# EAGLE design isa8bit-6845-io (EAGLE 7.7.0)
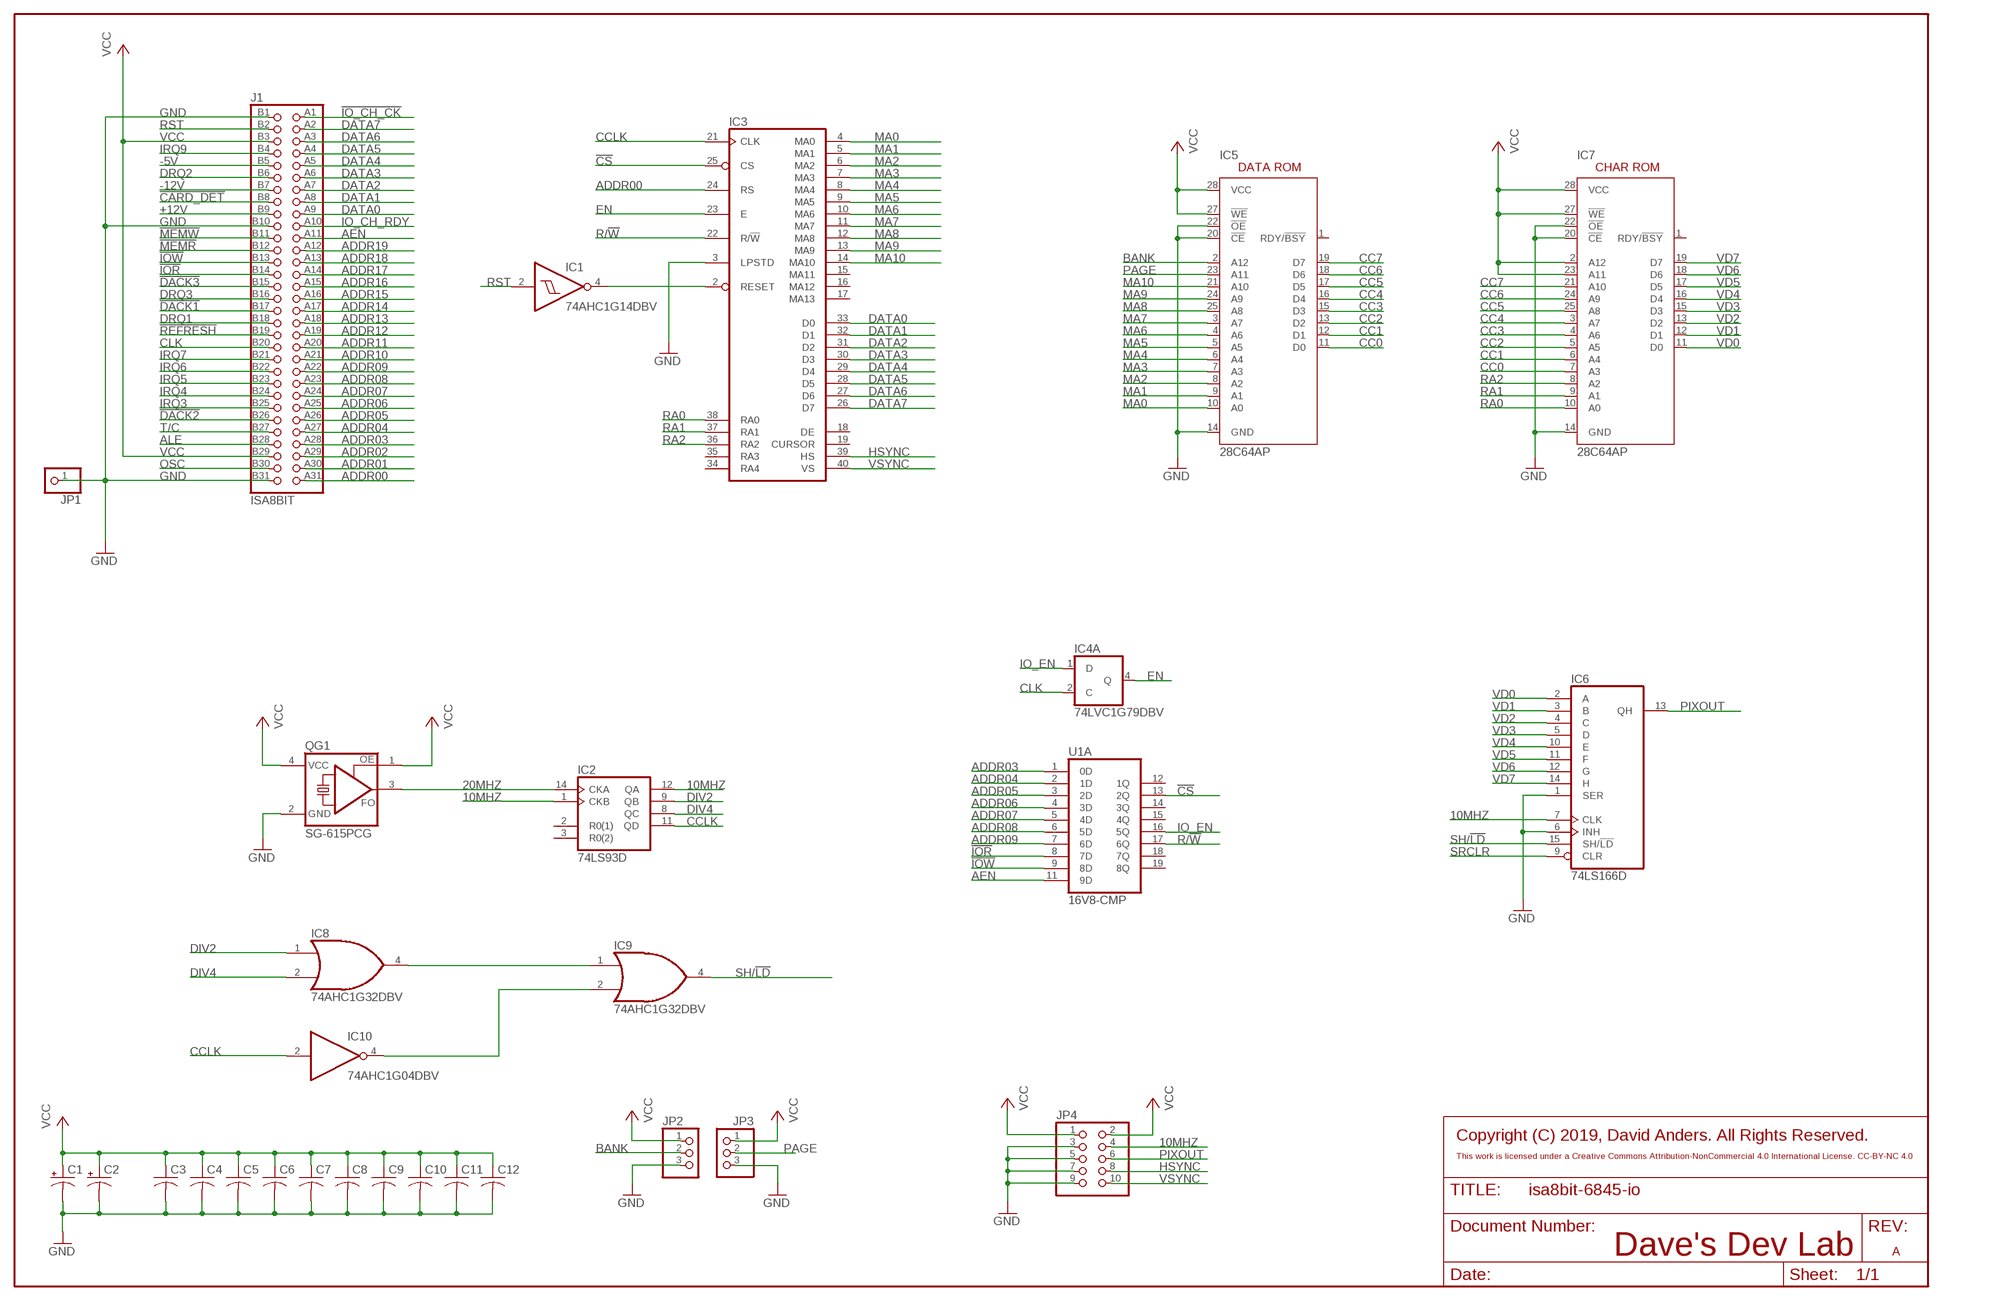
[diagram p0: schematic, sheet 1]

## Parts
C1  CPOL-USTT2D5  [TT2D5]
C2  CPOL-USTT2D5  [TT2D5]
C3  C-USC0603  [C0603]
C4  C-USC0603  [C0603]
C5  C-USC0603  [C0603]
C6  C-USC0603  [C0603]
C7  C-USC0603  [C0603]
C8  C-USC0603  [C0603]
C9  C-USC0603  [C0603]
C10  C-USC0603  [C0603]
C11  C-USC0603  [C0603]
C12  C-USC0603  [C0603]
IC1  74AHC1G14DBV  [SOT23-5]
IC2  74LS93D  [SO14]
IC3  6845  [DIL40]
IC4  74LVC1G79DBV  [SOT23-5]
IC5  28C64AP  [DIL28-6]
IC6  74LS166D  [SO16]
IC7  28C64AP  [DIL28-6]
IC8  74AHC1G32DBV  [SOT23-5]
IC9  74AHC1G32DBV  [SOT23-5]
IC10  74AHC1G04DBV  [SOT23-5]
J1  ISA8BIT  [ISA8BIT-LARGE]
JP1  PINHD-1X1  [1X01]
JP2  PINHD-1X3  [1X03]
JP3  PINHD-1X3  [1X03]
JP4  PINHD-2X5  [2X05]
QG1  SG-615PCG  [SG-615]
U1  16V8-CMP  [DIL20]

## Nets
10MHZ: IC2.1(CKB) IC2.12(QA) IC6.7(CLK) JP4.4
20MHZ: IC2.14(CKA) QG1.3(FO)
!CARD_DET: J1.B8
!CS: IC3.25(CS) U1.13(A:2Q)
!DACK1: J1.B17
!DACK2: J1.B26
!DACK3: J1.B15
!IO_CH_CK: J1.A1
!IOR: J1.B14 U1.8(A:7D)
!IOW: J1.B13 U1.9(A:8D)
!MEMR: J1.B12
!MEMW: J1.B11
!REFRESH: J1.B19
+12V: J1.B9
-5V: J1.B5
-12V: J1.B7
ADDR00: IC3.24(RS) J1.A31
ADDR01: J1.A30
ADDR02: J1.A29
ADDR03: J1.A28 U1.1(A:0D)
ADDR04: J1.A27 U1.2(A:1D)
ADDR05: J1.A26 U1.3(A:2D)
ADDR06: J1.A25 U1.4(A:3D)
ADDR07: J1.A24 U1.5(A:4D)
ADDR08: J1.A23 U1.6(A:5D)
ADDR09: J1.A22 U1.7(A:6D)
ADDR10: J1.A21
ADDR11: J1.A20
ADDR12: J1.A19
ADDR13: J1.A18
ADDR14: J1.A17
ADDR15: J1.A16
ADDR16: J1.A15
ADDR17: J1.A14
ADDR18: J1.A13
ADDR19: J1.A12
AEN: J1.A11 U1.11(A:9D)
ALE: J1.B28
BANK: IC5.2(A12) JP2.2
CC0: IC5.11(D0) IC7.7(A3)
CC1: IC5.12(D1) IC7.6(A4)
CC2: IC5.13(D2) IC7.5(A5)
CC3: IC5.15(D3) IC7.4(A6)
CC4: IC5.16(D4) IC7.3(A7)
CC5: IC5.17(D5) IC7.25(A8)
CC6: IC5.18(D6) IC7.24(A9)
CC7: IC5.19(D7) IC7.21(A10)
CCLK: IC2.11(QD) IC3.21(CLK) IC10.2(I)
CLK: IC4.2(C) J1.B20
DATA0: IC3.33(D0) J1.A9
DATA1: IC3.32(D1) J1.A8
DATA2: IC3.31(D2) J1.A7
DATA3: IC3.30(D3) J1.A6
DATA4: IC3.29(D4) J1.A5
DATA5: IC3.28(D5) J1.A4
DATA6: IC3.27(D6) J1.A3
DATA7: IC3.26(D7) J1.A2
DIV2: IC2.9(QB) IC8.1(I0)
DIV4: IC2.8(QC) IC8.2(I1)
DRQ1: J1.B18
DRQ2: J1.B6
DRQ3: J1.B16
EN: IC3.23(E) IC4.4(Q)
GND: C1.- C2.- C3.2 C4.2 C5.2 C6.2 C7.2 C8.2 C9.2 C10.2 C11.2 C12.2 IC3.3(LPSTD) IC5.14(GND) IC5.20(!CE) IC5.22(!OE) IC6.1(SER) IC6.6(INH) IC7.14(GND) IC7.20(!CE) IC7.22(!OE) J1.B1 J1.B10 J1.B31 JP1.1 JP2.3 JP3.3 JP4.3 JP4.5 JP4.7 JP4.9 QG1.2(GND)
HSYNC: IC3.39(HS) JP4.8
IO_CH_RDY: J1.A10
IO_EN: IC4.1(D) U1.16(A:5Q)
IRQ3: J1.B25
IRQ4: J1.B24
IRQ5: J1.B23
IRQ6: J1.B22
IRQ7: J1.B21
IRQ9: J1.B4
MA0: IC3.4(MA0) IC5.10(A0)
MA1: IC3.5(MA1) IC5.9(A1)
MA2: IC3.6(MA2) IC5.8(A2)
MA3: IC3.7(MA3) IC5.7(A3)
MA4: IC3.8(MA4) IC5.6(A4)
MA5: IC3.9(MA5) IC5.5(A5)
MA6: IC3.10(MA6) IC5.4(A6)
MA7: IC3.11(MA7) IC5.3(A7)
MA8: IC3.12(MA8) IC5.25(A8)
MA9: IC3.13(MA9) IC5.24(A9)
MA10: IC3.14(MA10) IC5.21(A10)
N$1: IC8.4(O) IC9.1(I0)
N$2: IC1.4(O) IC3.2(RESET)
N$4: IC9.2(I1) IC10.4(O)
OSC: J1.B30
PAGE: IC5.23(A11) JP3.2
PIXOUT: IC6.13(QH) JP4.6
R/!W: IC3.22(R/!W) U1.17(A:6Q)
RA0: IC3.38(RA0) IC7.10(A0)
RA1: IC3.37(RA1) IC7.9(A1)
RA2: IC3.36(RA2) IC7.8(A2)
RST: IC1.2(I) J1.B2
SH/!LD: IC6.15(SH/!LD) IC9.4(O)
SRCLR: IC6.9(CLR)
T/C: J1.B27
VCC: C1.+ C2.+ C3.1 C4.1 C5.1 C6.1 C7.1 C8.1 C9.1 C10.1 C11.1 C12.1 IC5.27(!WE) IC5.28(VCC) IC7.2(A12) IC7.23(A11) IC7.27(!WE) IC7.28(VCC) J1.B3 J1.B29 JP2.1 JP3.1 JP4.1 JP4.2 QG1.1(OE) QG1.4(VCC)
VD0: IC6.2(A) IC7.11(D0)
VD1: IC6.3(B) IC7.12(D1)
VD2: IC6.4(C) IC7.13(D2)
VD3: IC6.5(D) IC7.15(D3)
VD4: IC6.10(E) IC7.16(D4)
VD5: IC6.11(F) IC7.17(D5)
VD6: IC6.12(G) IC7.18(D6)
VD7: IC6.14(H) IC7.19(D7)
VSYNC: IC3.40(VS) JP4.10
Unconnected: IC2.2(R0(1)) IC2.3(R0(2)) IC3.15(MA11) IC3.16(MA12) IC3.17(MA13) IC3.18(DE) IC3.19(CURSOR) IC3.34(RA4) IC3.35(RA3) IC5.1(RDY/!BSY) IC7.1(RDY/!BSY) U1.12(A:1Q) U1.14(A:3Q) U1.15(A:4Q) U1.18(A:7Q) U1.19(A:8Q)

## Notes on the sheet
- DATA ROM | CHAR ROM
- Copyright (C) 2019, David Anders. All Rights Reserved.
- This work is licensed under a Creative Commons Attribution-NonCommercial 4.0 International License. CC-BY-NC 4.0
- Dave's Dev Lab | A

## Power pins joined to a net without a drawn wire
GND: IC1.3(GND) IC2.10(GND) IC3.1(GND) IC4.3(GND) IC6.8(GND) IC8.3(GND) IC9.3(GND) IC10.3(GND) U1.10(B:GND)
VCC: IC1.5(VCC) IC2.5(VCC) IC3.20(VCC) IC4.5(VCC) IC6.16(VCC) IC8.5(VCC) IC9.5(VCC) IC10.5(VCC) U1.20(B:VCC)

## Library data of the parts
C1 C2 = resistor:CPOL-US: POLARIZED CAPACITOR, American symbol
C3-C12 = resistor:C-US: CAPACITOR, American symbol
IC1 = 74xx-little-us:74*1G14: Single Schmitt-Trigger Inverter Gate
IC2 = 74xx-us:74*93: Decade, divide by twelve and binary COUNTER
IC3 = micro-motorola:6845: MICROCONTROLLER/MEMORY DEVICE; OC_FARNELL: unknown; OC_NEWARK: unknown
IC4 = 74xx-little-us:74*1G79: Single Positive-Edge-Triggered D-Type Flip-Flop Source: Data sheet
IC5 IC7 = microchip:28*64A: CMOS EEPROM 64 K (8 K x 8), low voltage; MPN: AT28C64B-15PU; OC_FARNELL: 1631144; OC_NEWARK: 96K6557
IC6 = 74xx-us:74*166: 8-bit parallel load SHIFT REGISTER
IC8 IC9 = 74xx-little-us:74*1G32: 2-input OR gate
IC10 = 74xx-little-us:74*1G04: INVERTER Gate
J1 = custom-misc:ISA8BIT
JP1 = custom-pinhead:PINHD-1X1: PIN HEADER
JP2 JP3 = custom-pinhead:PINHD-1X3: PIN HEADER
JP4 = custom-pinhead:PINHD-2X5: PIN HEADER
QG1 = crystal:SG-615: SOJ HIGH-FREQUENCY CRYSTAL OSCILLATOR Source: Crystal Oscillator SG-615%20Series.pdf; MPN: SG615P-50MHZ 50PPM; OC_FARNELL: 1216207; OC_NEWARK: 01M8855
U1 = custom-misc:16V8-CMP

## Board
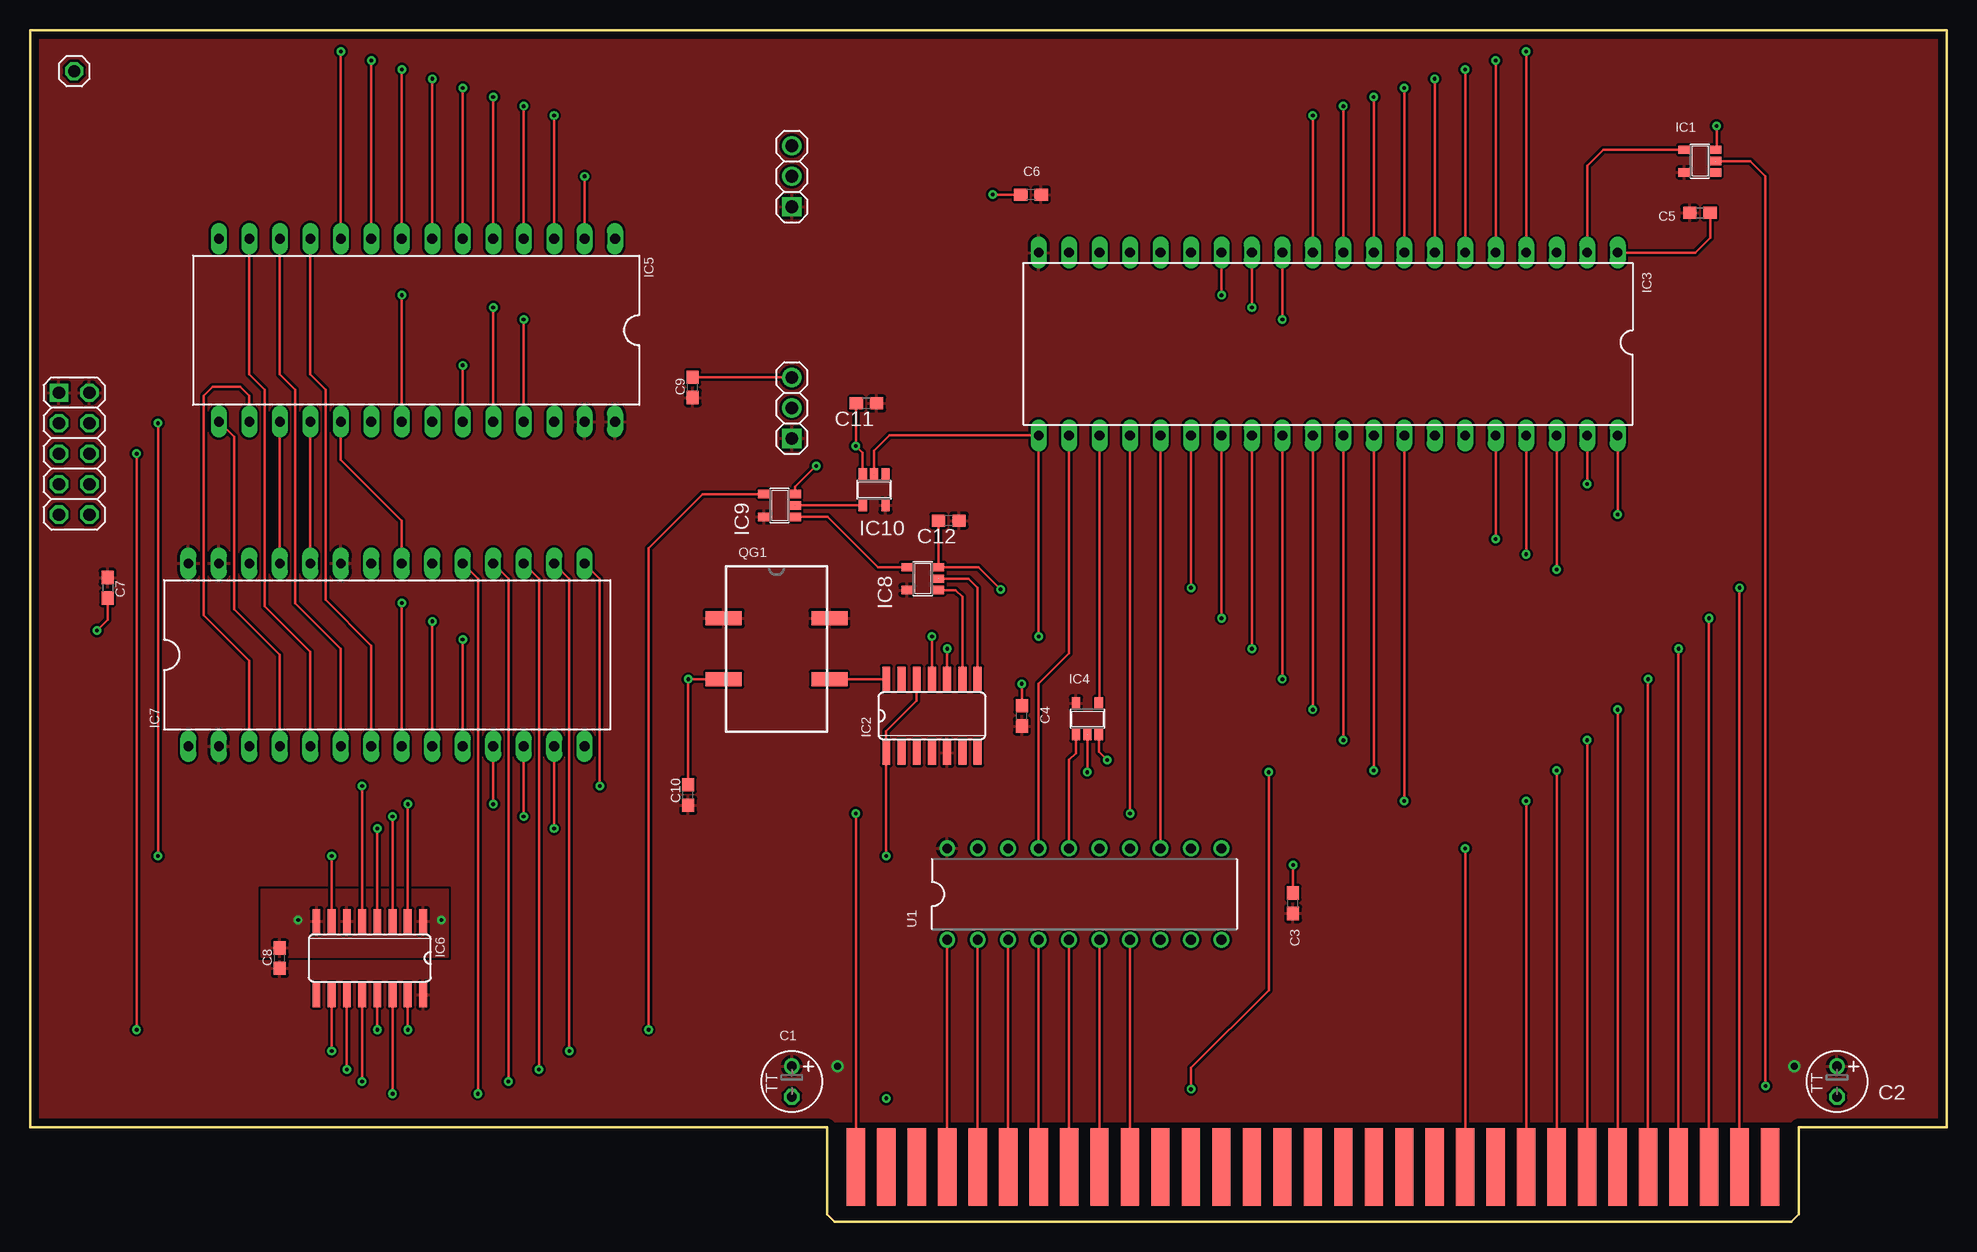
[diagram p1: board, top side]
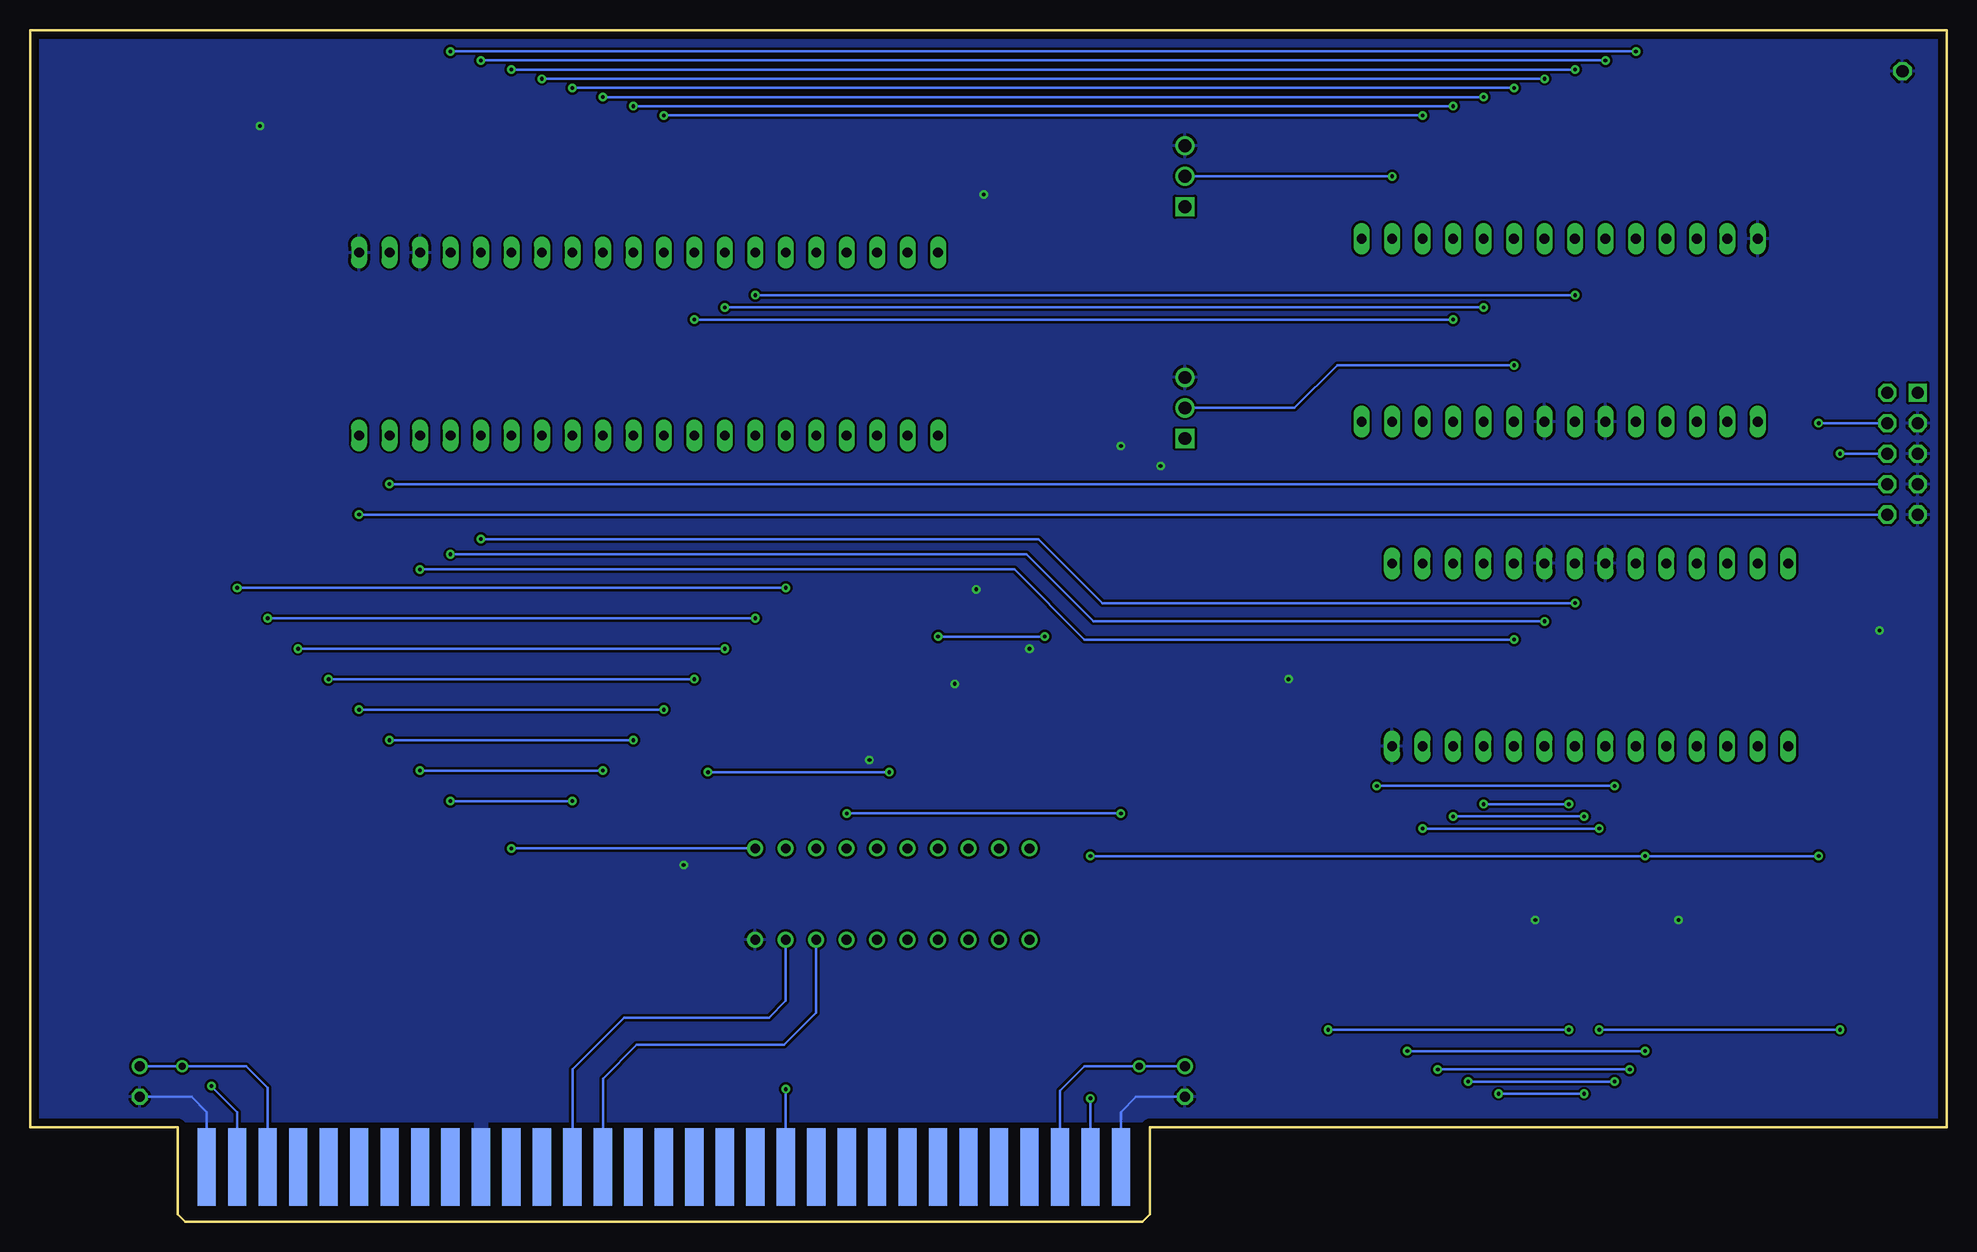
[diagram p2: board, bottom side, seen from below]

Size 159.77 x 99.31 mm. Coordinates in mm from the lower left corner, seen from the top.
Copper layers (1*16): Top 0.035mm / dielectric 1.5mm / Bottom 0.035mm
Design rules "default *": minimum track width 8mil, minimum drill 12mil, track to track 8mil, track to pad 8mil, pad to pad 8mil, via to via 8mil, smd to smd 8mil, copper to edge 25mil, drill to drill 8mil, minimum pad ring 10mil, minimum via ring 8mil, stop-mask expansion 4mil, vias tented up to drill 0mil, thermal gap 10mil

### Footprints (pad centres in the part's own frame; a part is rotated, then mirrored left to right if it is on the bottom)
TT2D5 = drill 0.813: + -1.27,0 | drill 0.813 octagon: - 1.27,0
C0603 = smd 1.1 x 1: 1 -0.85,0; 2 0.85,0
SOT23-5 = smd 0.69 x 0.99: 1 -0.95,-1.29; 2 0,-1.29; 3 0.95,-1.29; 4 0.95,1.3; 5 -0.95,1.3
SO14 = smd 0.66 x 2.032: 1 -3.81,-3.073; 2 -2.54,-3.073; 3 -1.27,-3.073; 4 0,-3.073; 5 1.27,-3.073; 6 2.54,-3.073; 7 3.81,-3.073; 8 3.81,3.073; 9 2.54,3.073; 10 1.27,3.073; 11 0,3.073; 12 -1.27,3.073; 13 -2.54,3.073; 14 -3.81,3.073
DIL40 = drill 0.813 long: 1 -24.13,-7.62; 2 -21.59,-7.62; 3 -19.05,-7.62; 4 -16.51,-7.62; 5 -13.97,-7.62; 6 -11.43,-7.62; 7 -8.89,-7.62; 8 -6.35,-7.62; 9 -3.81,-7.62; 10 -1.27,-7.62; 11 1.27,-7.62; 12 3.81,-7.62; 13 6.35,-7.62; 14 8.89,-7.62; 15 11.43,-7.62; 16 13.97,-7.62; 17 16.51,-7.62; 18 19.05,-7.62; 19 21.59,-7.62; 20 24.13,-7.62; 21 24.13,7.62; 22 21.59,7.62; 23 19.05,7.62; 24 16.51,7.62; 25 13.97,7.62; 26 11.43,7.62; 27 8.89,7.62; 28 6.35,7.62; 29 3.81,7.62; 30 1.27,7.62; 31 -1.27,7.62; 32 -3.81,7.62; 33 -6.35,7.62; 34 -8.89,7.62; 35 -11.43,7.62; 36 -13.97,7.62; 37 -16.51,7.62; 38 -19.05,7.62; 39 -21.59,7.62; 40 -24.13,7.62
DIL28-6 = drill 0.813 long: 1 -16.51,-7.62; 2 -13.97,-7.62; 3 -11.43,-7.62; 4 -8.89,-7.62; 5 -6.35,-7.62; 6 -3.81,-7.62; 7 -1.27,-7.62; 8 1.27,-7.62; 9 3.81,-7.62; 10 6.35,-7.62; 11 8.89,-7.62; 12 11.43,-7.62; 13 13.97,-7.62; 14 16.51,-7.62; 15 16.51,7.62; 16 13.97,7.62; 17 11.43,7.62; 18 8.89,7.62; 19 6.35,7.62; 20 3.81,7.62; 21 1.27,7.62; 22 -1.27,7.62; 23 -3.81,7.62; 24 -6.35,7.62; 25 -8.89,7.62; 26 -11.43,7.62; 27 -13.97,7.62; 28 -16.51,7.62
SO16 = smd 0.66 x 2.032: 1 -4.445,-3.073; 2 -3.175,-3.073; 3 -1.905,-3.073; 4 -0.635,-3.073; 5 0.635,-3.073; 6 1.905,-3.073; 7 3.175,-3.073; 8 4.445,-3.073; 9 4.445,3.073; 10 3.175,3.073; 11 1.905,3.073; 12 0.635,3.073; 13 -0.635,3.073; 14 -1.905,3.073; 15 -3.175,3.073; 16 -4.445,3.073
ISA8BIT-LARGE = smd 1.524 x 6.477: A1 145.034,5.08; A2 142.494,5.08; A3 139.954,5.08; A4 137.414,5.08; A5 134.874,5.08; A6 132.334,5.08; A7 129.794,5.08; A8 127.254,5.08; A9 124.714,5.08; A10 122.174,5.08; A11 119.634,5.08; A12 117.094,5.08; A13 114.554,5.08; A14 112.014,5.08; A15 109.474,5.08; A16 106.934,5.08; A17 104.394,5.08; A18 101.854,5.08; A19 99.314,5.08; A20 96.774,5.08; A21 94.234,5.08; A22 91.694,5.08; A23 89.154,5.08; A24 86.614,5.08; A25 84.074,5.08; A26 81.534,5.08; A27 78.994,5.08; A28 76.454,5.08; A29 73.914,5.08; A30 71.374,5.08; A31 68.834,5.08 | smd 1.524 x 6.477 bottom: B1 145.034,5.08; B2 142.494,5.08; B3 139.954,5.08; B4 137.414,5.08; B5 134.874,5.08; B6 132.334,5.08; B7 129.794,5.08; B8 127.254,5.08; B9 124.714,5.08; B10 122.174,5.08; B11 119.634,5.08; B12 117.094,5.08; B13 114.554,5.08; B14 112.014,5.08; B15 109.474,5.08; B16 106.934,5.08; B17 104.394,5.08; B18 101.854,5.08; B19 99.314,5.08; B20 96.774,5.08; B21 94.234,5.08; B22 91.694,5.08; B23 89.154,5.08; B24 86.614,5.08; B25 84.074,5.08; B26 81.534,5.08; B27 78.994,5.08; B28 76.454,5.08; B29 73.914,5.08; B30 71.374,5.08; B31 68.834,5.08
1X01 = drill 1.016 octagon: 1 0,0
1X03 = drill 1.067 square: 1 -2.54,0 | drill 1.067: 2 0,0; 3 2.54,0
2X05 = drill 1.016 square: 1 -5.08,-1.27 | drill 1.016 octagon: 2 -5.08,1.27; 3 -2.54,-1.27; 4 -2.54,1.27; 5 0,-1.27; 6 0,1.27; 7 2.54,-1.27; 8 2.54,1.27; 9 5.08,-1.27; 10 5.08,1.27
SG-615 = smd 1.2 x 3: 1 -2.54,-4.4; 2 2.54,-4.4; 3 2.54,4.4; 4 -2.54,4.4
DIL20 = drill 0.813: 1 -11.43,-3.81; 2 -8.89,-3.81; 3 -6.35,-3.81; 4 -3.81,-3.81; 5 -1.27,-3.81; 6 1.27,-3.81; 7 3.81,-3.81; 8 6.35,-3.81; 9 8.89,-3.81; 10 11.43,-3.81; 11 11.43,3.81; 12 8.89,3.81; 13 6.35,3.81; 14 3.81,3.81; 15 1.27,3.81; 16 -1.27,3.81; 17 -3.81,3.81; 18 -6.35,3.81; 19 -8.89,3.81; 20 -11.43,3.81

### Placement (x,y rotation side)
C1  63.5,11.68 270 top
C2  150.62,11.68 270 top
C3  105.28,26.54 90 top
C4  82.68,42.16 90 top
C5  139.19,84.07 0 top
C6  83.44,85.6 180 top
C7  6.48,52.83 270 top
C8  20.83,21.97 90 top
C9  55.24,69.53 90 top
C10  54.86,35.56 90 top
C11  69.72,68.2 180 top
C12  76.58,58.42 180 top
IC1  139.19,88.39 90 top
IC2  75.18,42.16 0 top
IC3  108.2,73.15 180 top
IC4  88.14,41.91 0 top
IC5  32.26,74.3 180 top
IC6  28.32,21.97 180 top
IC7  29.72,47.24 0 top
IC8  74.42,53.59 90 top
IC9  62.48,59.69 90 top
IC10  70.36,61 180 top
J1  0,-0.51 0 top
JP1  3.68,95.89 0 top
JP2  63.5,87.12 90 top
JP3  63.5,67.82 90 top
JP4  3.68,64.01 270 top
QG1  62.23,47.75 270 top
U1  87.88,27.3 0 top

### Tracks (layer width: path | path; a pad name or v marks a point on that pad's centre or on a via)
10MHZ  (via drill 0.3)
  Top 0.203: IC2.12 73.91,43.43 71.37,40.89 IC2.1 v71.37,30.48 | IC6.7 v25.15,30.48 | v10.67,30.48 v10.67,66.55
  Bottom 0.203: v71.37,30.48 v25.15,30.48 v10.67,30.48 | v10.67,66.55 JP4.4
20MHZ
  Top 0.203: QG1.3 71.35,45.21 IC2.14
!CS
  Top 0.203: IC3.25 U1.13
!IOR
  Bottom 0.203: U1.8 94.23,17.4 96.9,14.73 109.22,14.73 112.01,11.94 J1.B14
!IOW
  Bottom 0.203: U1.9 96.77,18.41 98.17,17.02 110.24,17.02 114.55,12.7 J1.B13
ADDR00  (via drill 0.3)
  Top 0.203: J1.A31 v68.83,34.04 | v91.69,34.04 IC3.24
  Bottom 0.203: v68.83,34.04 v91.69,34.04
ADDR03
  Top 0.203: J1.A28 U1.1
ADDR04
  Top 0.203: J1.A27 U1.2
ADDR05
  Top 0.203: J1.A26 U1.3
ADDR06
  Top 0.203: J1.A25 U1.4
ADDR07
  Top 0.203: J1.A24 U1.5
ADDR08
  Top 0.203: J1.A23 U1.6
ADDR09
  Top 0.203: J1.A22 U1.7
AEN  (via drill 0.3)
  Top 0.203: J1.A11 v119.63,31.12
  Bottom 0.203: v119.63,31.12 U1.11
BANK  (via drill 0.3)
  Top 0.203: IC5.2 v46.23,87.12
  Bottom 0.203: v46.23,87.12 JP2.2
CC0
  Top 0.203: IC7.7 28.45,48.01 24.64,51.82 24.64,69.34 23.37,70.61 IC5.11
CC1
  Top 0.203: IC7.6 25.91,47.75 22.1,51.56 22.1,69.34 20.83,70.61 IC5.12
CC2
  Top 0.203: IC7.5 23.37,47.5 19.56,51.31 19.56,69.34 18.29,70.61 IC5.13
CC3
  Top 0.203: IC5.15 17.02,65.41 17.02,51.05 20.83,47.24 IC7.4
CC4
  Top 0.203: IC7.3 18.29,46.74 14.48,50.55 14.48,68.83 15.24,69.6 17.53,69.6 18.29,68.83 IC5.16
CC5
  Top 0.203: IC5.17 IC7.25
CC6
  Top 0.203: IC5.18 IC7.24
CC7
  Top 0.203: IC5.19 25.91,63.5 30.99,58.42 IC7.21
CCLK  (via drill 0.3)
  Top 0.203: IC10.2 70.36,64.26 71.63,65.53 IC3.21 v84.07,48.77 | IC2.11 v75.18,48.77
  Bottom 0.203: v75.18,48.77 v84.07,48.77
CLK  (via drill 0.3)
  Top 0.203: v96.77,11.05 96.77,12.83 103.25,19.3 v103.25,37.46 | v88.14,37.46 IC4.2
  Bottom 0.203: J1.B20 v96.77,11.05 | v103.25,37.46 v88.14,37.46
DATA0  (via drill 0.3)
  Top 0.203: J1.A9 v124.71,35.05 | v114.55,35.05 IC3.33
  Bottom 0.203: v124.71,35.05 v114.55,35.05
DATA1  (via drill 0.3)
  Top 0.203: J1.A8 v127.25,37.59 | v112.01,37.59 IC3.32
  Bottom 0.203: v127.25,37.59 v112.01,37.59
DATA2  (via drill 0.3)
  Top 0.203: J1.A7 v129.79,40.13 | v109.47,40.13 IC3.31
  Bottom 0.203: v129.79,40.13 v109.47,40.13
DATA3  (via drill 0.3)
  Top 0.203: J1.A6 v132.33,42.67 | v106.93,42.67 IC3.30
  Bottom 0.203: v132.33,42.67 v106.93,42.67
DATA4  (via drill 0.3)
  Top 0.203: IC3.29 v104.39,45.21 | J1.A5 v134.87,45.21
  Bottom 0.203: v104.39,45.21 v134.87,45.21
DATA5  (via drill 0.3)
  Top 0.203: IC3.28 v101.85,47.75 | J1.A4 v137.41,47.75
  Bottom 0.203: v137.41,47.75 v101.85,47.75
DATA6  (via drill 0.3)
  Top 0.203: IC3.27 v99.31,50.29 | J1.A3 v139.95,50.29
  Bottom 0.203: v139.95,50.29 v99.31,50.29
DATA7  (via drill 0.3)
  Top 0.203: IC3.26 v96.77,52.83 | v142.49,52.83 J1.A2
  Bottom 0.203: v96.77,52.83 v142.49,52.83
DIV2
  Top 0.203: IC8.1 77.15,52.64 77.72,52.07 IC2.9
DIV4
  Top 0.203: IC2.8 78.99,52.83 78.23,53.59 IC8.2
EN
  Top 0.203: IC4.4 89.15,43.28 IC3.23
GND  (via drill 0.3)
  Top 0.203: IC3.1 138.81,80.77 140.04,82 C5.2 | IC1.3 140.59,89.45 v140.59,91.31 | C3.2 v105.28,29.72 | IC4.3 89.09,39.18 v89.79,38.48 | C6.2 v80.26,85.6 | QG1.2 v54.86,45.21 C10.2 | C9.2 63.48,70.38 JP3.3 | C7.2 6.48,50.16 v5.59,49.28 | IC2.10 v76.45,47.75 | C4.2 v82.68,44.83 | IC9.3 63.77,61.23 v65.53,62.99 | IC10.3 69.41,64.07 v68.83,64.64 68.87,64.68 C11.2 | C12.2 75.71,58.4 IC8.3 79.06,54.54 v80.9,52.7
  Bottom 0.203: C1.- 67.56,10.41 68.83,9.14 J1.B31 | J1.B1 145.03,9.14 146.3,10.41 C2.-
  other vias: 22.35,25.15 34.29,25.15
  pour Bottom: 0,8.38 0,99.31 159.77,99.31 159.77,8.38
  pour Bottom (no thermals): 121.67,3.3 121.67,8.38 122.68,8.38 122.68,3.3
  pour Top: 19.3,27.69 19.3,22.1 34.8,22.1 34.8,27.69
HSYNC  (via drill 0.3)
  Top 0.203: v129.79,61.47 IC3.39
  Bottom 0.203: JP4.8 v129.79,61.47
IO_EN
  Top 0.203: U1.16 86.61,38.48 87.19,39.05 IC4.1
MA0  (via drill 0.3)
  Top 0.203: IC3.4 v124.71,97.54 | v25.91,97.54 IC5.10
  Bottom 0.203: v124.71,97.54 v25.91,97.54
MA1  (via drill 0.3)
  Top 0.203: IC5.9 v28.45,96.77 | v122.17,96.77 IC3.5
  Bottom 0.203: v28.45,96.77 v122.17,96.77
MA2  (via drill 0.3)
  Top 0.203: IC5.8 v30.99,96.01 | v119.63,96.01 IC3.6
  Bottom 0.203: v30.99,96.01 v119.63,96.01
MA3  (via drill 0.3)
  Top 0.203: IC5.7 v33.53,95.25 | v117.09,95.25 IC3.7
  Bottom 0.203: v33.53,95.25 v117.09,95.25
MA4  (via drill 0.3)
  Top 0.203: IC5.6 v36.07,94.49 | v114.55,94.49 IC3.8
  Bottom 0.203: v36.07,94.49 v114.55,94.49
MA5  (via drill 0.3)
  Top 0.203: IC5.5 v38.61,93.73 | v112.01,93.73 IC3.9
  Bottom 0.203: v38.61,93.73 v112.01,93.73
MA6  (via drill 0.3)
  Top 0.203: IC5.4 v41.15,92.96 | v109.47,92.96 IC3.10
  Bottom 0.203: v41.15,92.96 v109.47,92.96
MA7  (via drill 0.3)
  Top 0.203: IC5.3 v43.69,92.2 | v106.93,92.2 IC3.11
  Bottom 0.203: v43.69,92.2 v106.93,92.2
MA8  (via drill 0.3)
  Top 0.203: IC3.12 v104.39,75.18 | v41.15,75.18 IC5.25
  Bottom 0.203: v104.39,75.18 v41.15,75.18
MA9  (via drill 0.3)
  Top 0.203: IC3.13 v101.85,76.2 | v38.61,76.2 IC5.24
  Bottom 0.203: v101.85,76.2 v38.61,76.2
MA10  (via drill 0.3)
  Top 0.203: IC3.14 v99.31,77.22 | v30.99,77.22 IC5.21
  Bottom 0.203: v99.31,77.22 v30.99,77.22
N$1
  Top 0.203: IC9.1 66.48,58.74 70.68,54.54 IC8.4
N$2
  Top 0.203: IC1.4 131.12,89.34 129.79,88.01 IC3.2
N$4
  Top 0.203: IC9.2 63.78,59.7 IC10.4
OSC  (via drill 0.3)
  Bottom 0.203: J1.B30 v71.37,10.29
PAGE  (via drill 0.3)
  Top 0.203: IC5.23 v36.07,71.37
  Bottom 0.203: v36.07,71.37 50.8,71.37 54.36,67.82 JP3.2
PIXOUT  (via drill 0.3)
  Top 0.203: IC6.13 v28.96,16 | v8.89,16 v8.89,64.01
  Bottom 0.203: v28.96,16 v8.89,16 | v8.89,64.01 JP4.6
R/!W
  Top 0.203: U1.17 84.07,44.83 86.61,47.37 IC3.22
RA0  (via drill 0.3)
  Top 0.203: IC7.10 v36.07,48.51 | v127.25,54.36 IC3.38
  Bottom 0.203: v36.07,48.51 71.88,48.51 77.72,54.36 v127.25,54.36
RA1  (via drill 0.3)
  Top 0.203: IC7.9 v33.53,50.04 | v124.71,55.63 IC3.37
  Bottom 0.203: v33.53,50.04 71.12,50.04 76.71,55.63 v124.71,55.63
RA2  (via drill 0.3)
  Top 0.203: IC7.8 v30.99,51.56 | v122.17,56.9 IC3.36
  Bottom 0.203: v30.99,51.56 70.36,51.56 75.69,56.9 v122.17,56.9
RST  (via drill 0.3)
  Top 0.203: v144.65,11.3 144.65,87.12 143.38,88.39 IC1.2
  Bottom 0.203: J1.B2 142.49,9.14 v144.65,11.3
SH/!LD  (via drill 0.3)
  Top 0.203: IC6.15 v31.5,16 | v51.56,16 51.56,56.13 56.07,60.64 IC9.4
  Bottom 0.203: v31.5,16 v51.56,16
VCC  (via drill 0.6)
  Bottom 0.203: J1.B29 73.91,10.92 71.88,12.95 v67.31,12.95 C1.+ | J1.B3 139.95,11.18 141.73,12.95 v147.07,12.95 C2.+
  pour Top (rank 6): 0,8.38 0,99.31 159.77,99.31 159.77,8.38
VD0  (via drill 0.3)
  Top 0.203: IC7.11 v38.61,34.8 | v31.5,34.8 IC6.2
  Bottom 0.203: v38.61,34.8 v31.5,34.8
VD1  (via drill 0.3)
  Top 0.203: IC7.12 v41.15,33.78 | v30.23,33.78 IC6.3
  Bottom 0.203: v41.15,33.78 v30.23,33.78
VD2  (via drill 0.3)
  Top 0.203: IC7.13 v43.69,32.77 | v28.96,32.77 IC6.4
  Bottom 0.203: v43.69,32.77 v28.96,32.77
VD3  (via drill 0.3)
  Top 0.203: IC7.15 47.5,53.59 v47.5,36.32 | v27.69,36.32 IC6.5
  Bottom 0.203: v47.5,36.32 v27.69,36.32
VD4  (via drill 0.3)
  Top 0.203: IC7.16 44.96,53.59 v44.96,14.22 | v25.15,14.22 IC6.10
  Bottom 0.203: v44.96,14.22 v25.15,14.22
VD5  (via drill 0.3)
  Top 0.203: IC7.17 42.42,53.59 v42.42,12.7 | v26.42,12.7 IC6.11
  Bottom 0.203: v42.42,12.7 v26.42,12.7
VD6  (via drill 0.3)
  Top 0.203: IC7.18 39.88,53.59 v39.88,11.68 | v27.69,11.68 IC6.12
  Bottom 0.203: v39.88,11.68 v27.69,11.68
VD7  (via drill 0.3)
  Top 0.203: IC7.19 37.34,53.59 v37.34,10.67 | v30.23,10.67 IC6.14
  Bottom 0.203: v37.34,10.67 v30.23,10.67
VSYNC  (via drill 0.3)
  Top 0.203: v132.33,58.93 IC3.40
  Bottom 0.203: JP4.10 v132.33,58.93

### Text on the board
Document: GND | BANK | PAGE | Revision A | 8-BIT ISA MC6845 Video Test Board
tDocu: Copyright (C) 2019, David Anders. All Rights Reserved. | This work is licensed under a / Creative Commons Attribution-NonCommercial 4.0 International License. / CC-BY-NC 4.0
